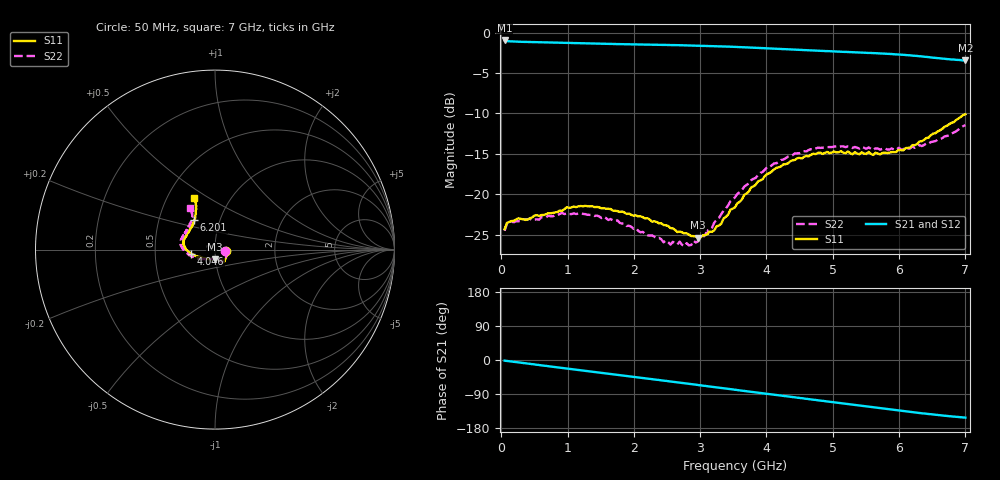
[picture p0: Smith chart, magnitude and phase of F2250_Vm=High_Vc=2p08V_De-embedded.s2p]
! Integrated Device Technology
! Corporate Headquarters
! 6024 Silver Creek Valley Road
! San Jose, CA 95138  USA
! Phone:  1-408-284-8200
! Toll Free:  1-800-223-1366
! Webpage:  http://www.idt.com/
! Timing and RF Division
! 515 Groton Road, Suite 102
! Westford, MA 01886-6024
! Device:  F2250
! Description: Voltage Variable RF Attenuator
! Frequency:  50.0 -  6000.00 MHz
! Package:  3x3 mm Thin QFN Plastic Package: 16 pin
! Ports:  2 RF, 3 DC
!  Pin  1  = GND
!  Pin  2  = NC
!  Pin  3  = RF1  = Port 1
!  Pin  4  = NC
!  Pin  5  = GND
!  Pin  6  = GND
!  Pin  7  = GND
!  Pin  8  = GND
!  Pin  9  = NC
!  Pin 10  = RF2  = Port 2
!  Pin 11  = NC
!  Pin 12  = GND
!  Pin 13  = GND
!  Pin 14  = VCNTRL
!  Pin 15  = VDD
!  Pin 16  = VMODE
! Vcntrl:  2.080 Volts
! Vmode:  +3.300 Volts
! Vdd:  +3.30  Volts
! Current:  1.319 mA
! Data:  The device was measured on a the F2250 evaluation board which has
!  individual transmission lines to the RF pins.  Data was collected
!  using a calibrated network analyzer.  The evaluation board was
!  de-embedded using a TRL calibration technique.
!  The reference plane is the edge of the package pin.
! Misc:  SN 10
!  Action Tracker AT0258
! Date Measured:  2014-11-26
! Date:  2015-10-15  MJV
! Note:
!  Integrated Device Technology supplies this data as a sample of measured
!  data at the package pin for this product.  Your particular data for this
!  product may vary.
!  Data was taken at 25 degrees C.
!  Integrated Device Technology reserves the right to change this data at anytime.
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# GHz S dB R 50
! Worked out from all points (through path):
!   201 points, 50 MHz to 7 GHz, reference 50 ohm
!   highest |S21| = -0.97 dB at 50 MHz (marker M1); lowest = -3.4 dB at 7 GHz (marker M2)
!   group delay of S21, straight-line fit = 61.1 ps
!   lowest |S11| = -25.4 dB at 2.969 GHz (marker M3), VSWR 1.11, Z = 49.7 - j5.36 ohm
!   |S11| at or under -10 dB: start of sweep to end of sweep
!   |S22| runs from -26.4 to -11.5 dB; largest |S21 - S12| = 0.0019
!   S11 on the Smith chart (normalised r, x): 50 MHz: 1.13, -0.02; 4.046 GHz: 0.76, -0.03; 6.201 GHz: 0.75, +0.26; 7 GHz: 0.68, +0.44
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0.05  -24.34 -9.2  -0.97 -1.8  -0.97 -1.8  -24.54 -9.8
0.08475  -23.56 -8.4  -1.05 -2.5  -1.04 -2.5  -23.64 -8.8
0.1195  -23.44 -9.0  -1.08 -3.3  -1.07 -3.2  -23.45 -8.2
0.91875  -22.07 -46.0  -1.26 -21.0  -1.26 -21.1  -22.34 -48.6
1.2315  -21.51 -53.7  -1.33 -27.9  -1.33 -27.9  -22.45 -59.0
1.75275  -22.09 -60.6  -1.42 -39.1  -1.42 -39.1  -23.25 -66.5
2.37825  -23.61 -61.0  -1.51 -52.8  -1.52 -52.8  -25.41 -68.9
2.552  -24.21 -65.3  -1.54 -56.6  -1.54 -56.6  -26.26 -75.5
2.691  -24.64 -72.4  -1.56 -59.7  -1.56 -59.7  -25.88 -82.6
2.7605  -24.86 -74.3  -1.58 -61.3  -1.58 -61.3  -26.44 -86.9
2.969  -25.40 -90.1  -1.61 -65.9  -1.61 -66.0  -25.84 -104.5
3.21225  -24.49 -119.3  -1.67 -71.4  -1.67 -71.5  -23.53 -128.1
3.525  -21.64 -146.5  -1.77 -78.5  -1.77 -78.5  -20.39 -146.8
3.76825  -19.17 -160.2  -1.86 -84.0  -1.86 -84.0  -18.29 -158.1
4.04625  -17.40 -170.4  -1.97 -90.2  -1.97 -90.2  -16.63 -168.7
4.4285  -15.76 178.9  -2.12 -98.6  -2.12 -98.6  -14.96 179.7
4.7065  -14.99 171.7  -2.22 -104.8  -2.22 -104.8  -14.47 173.8
5.054  -14.84 163.4  -2.35 -112.4  -2.34 -112.5  -14.07 166.6
5.85325  -14.88 137.3  -2.64 -129.9  -2.64 -130.1  -14.48 147.7
6.20075  -13.92 125.3  -2.85 -137.7  -2.85 -137.7  -14.08 138.6
6.54825  -12.45 117.0  -3.12 -144.7  -3.12 -144.8  -13.44 127.2
7  -10.11 111.9  -3.45 -152.0  -3.46 -152.1  -11.45 120.9
